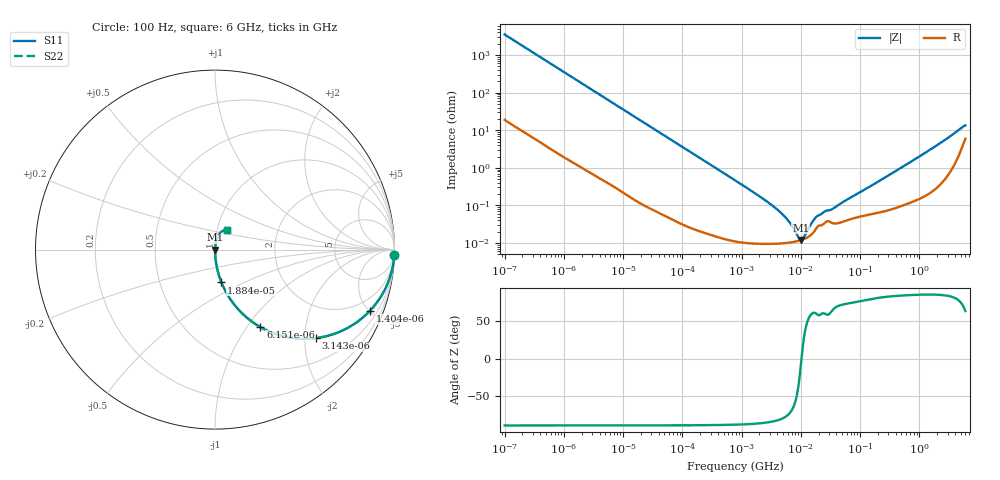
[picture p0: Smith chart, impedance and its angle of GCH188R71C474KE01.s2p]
!Murata Part Number: GCH188R71C474KE01
!These Parameters are Measured in Series Mode Connection
!Data Generated on Jun 19, 2026
!  o--ll--o
!Port1  Port2
!  o------o
!Operation Temp=25[degC], DC Bias Voltage=0[V]
!Freq. Start=100[Hz] Stop=6[GHz] 401[Steps]
# Hz S RI R 50
!Freq.(Hz) S11(Real) S11(Imag) S21(Real) S21(Imag) S12(Real) S12(Imag) S22(Real) S22(Imag)
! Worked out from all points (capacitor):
!   401 points, 100 Hz to 6 GHz, reference 50 ohm
!   read as one part in series: C = 452 nF near 109 Hz
!   lowest |Z| = 12.1 mohm at 9.942 MHz (marker M1)
!   series resonance near 10.28 MHz, so ESL is about 530 pH
!   S11 on the Smith chart (normalised r, x): 100 Hz: 1, -70; 1.404 kHz: 1.03, -5.05; 3.143 kHz: 1.01, -2.26; 6.151 kHz: 1.01, -1.16; 18.84 kHz: 1.00, -0.38; 6 GHz: 1.12, +0.24
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100  0.999 -0.0284  0.000961 0.0284  0.000961 0.0284  0.999 -0.0284
438  0.9842 -0.122  0.0158 0.122  0.0158 0.122  0.9842 -0.122
1404  0.8632 -0.3409  0.1368 0.3409  0.1368 0.3409  0.8632 -0.3409
2008  0.7565 -0.4264  0.2435 0.4264  0.2435 0.4264  0.7565 -0.4264
3143  0.5613 -0.4933  0.4387 0.4933  0.4387 0.4933  0.5613 -0.4933
6151  0.2529 -0.4316  0.7471 0.4316  0.7471 0.4316  0.2529 -0.4316
10066  0.1134 -0.3141  0.8866 0.3141  0.8866 0.3141  0.1134 -0.3141
18841  0.0359 -0.183  0.9641 0.183  0.9641 0.183  0.0359 -0.183
40335  0.00848 -0.0882  0.9915 0.0882  0.9915 0.0882  0.00848 -0.0882
774597  0.000132 -0.00467  0.9999 0.00467  0.9999 0.00467  0.000132 -0.00467
4246196  9.71e-05 -0.000712  0.9999 0.000712  0.9999 0.000712  9.71e-05 -0.000712
6353432  0.000102 -0.000355  0.9999 0.000355  0.9999 0.000355  0.000102 -0.000355
9090158  0.000114 -8.8e-05  0.9999 8.8e-05  0.9999 8.8e-05  0.000114 -8.8e-05
9941735  0.000119 -2.39e-05  0.9999 2.39e-05  0.9999 2.39e-05  0.000119 -2.39e-05
1.137099e7  0.000128 7.25e-05  0.9999 -7.25e-05  0.9999 -7.25e-05  0.000128 7.25e-05
1.555665e7  0.000176 0.000312  0.9998 -0.000312  0.9998 -0.000312  0.000176 0.000312
1.86079e7  0.000257 0.000441  0.9997 -0.000441  0.9997 -0.000441  0.000257 0.000441
2.434276e7  0.000323 0.000578  0.9997 -0.000578  0.9997 -0.000578  0.000323 0.000578
3.482834e7  0.000337 0.000746  0.9997 -0.000746  0.9997 -0.000746  0.000337 0.000746
3.124326e8  0.000797 0.00644  0.9992 -0.00644  0.9992 -0.00644  0.000797 0.00644
2.931063e9  0.00929 0.0588  0.9907 -0.0588  0.9907 -0.0588  0.00929 0.0588
6e9  0.0684 0.1064  0.9316 -0.1064  0.9316 -0.1064  0.0684 0.1064
